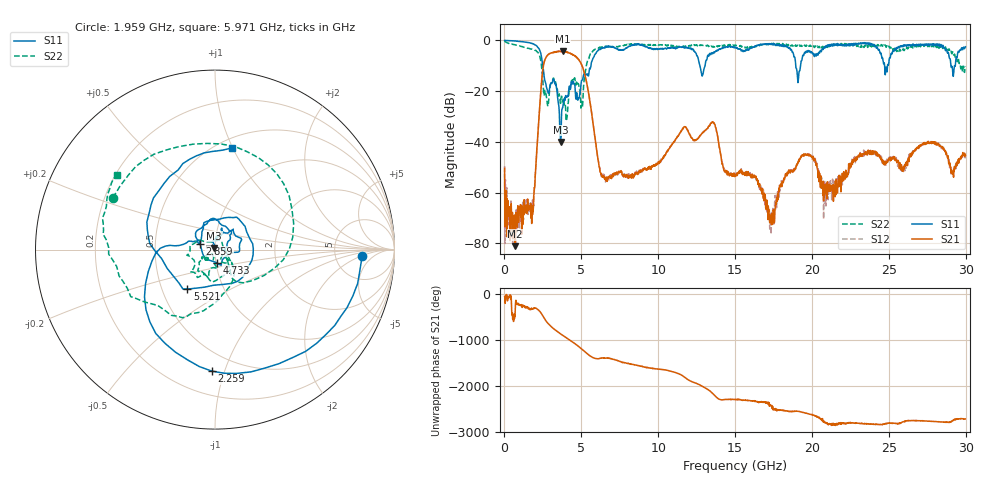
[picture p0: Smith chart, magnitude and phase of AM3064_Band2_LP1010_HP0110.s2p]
# Hz S DB R 50.0
!freq dBS11 angS11 dBS21 angS21 dBS12 angS12 dBS22 angS22
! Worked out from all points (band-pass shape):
!   1600 points, 10 MHz to 29.98 GHz, reference 50 ohm
!   highest |S21| = -4.27 dB at 3.777 GHz (marker M1); lowest = -81.1 dB at 703.5 MHz (marker M2)
!   |S21| within 3 dB of the highest: 2.656 GHz to 4.791 GHz (2.135 GHz wide, 57.3 % of centre)
!   lowest |S11| = -40.1 dB at 3.646 GHz (marker M3), VSWR 1.02, Z = 49.5 + j0.88 ohm
!   |S11| at or under -10 dB: 2.494 GHz to 5.622 GHz (3.129 GHz wide, 77.1 % of centre); 12.71 GHz to 13.05 GHz (331.7 MHz wide, 2.58 % of centre); 18.95 GHz to 19.25 GHz (303.6 MHz wide, 1.59 % of centre)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
!   |S22| runs from -31.2 to -0.3 dB; largest |S21 - S12| = 0.017
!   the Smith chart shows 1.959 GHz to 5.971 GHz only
!   S11 on the Smith chart (normalised r, x): 1.959 GHz: 9.63, -2.16; 2.259 GHz: 0.36, -0.91; 2.859 GHz: 0.84, +0.06; 4.733 GHz: 1.01, -0.15; 5.521 GHz: 0.67, -0.32; 5.971 GHz: 0.59, +0.99
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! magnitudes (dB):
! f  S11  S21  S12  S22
! 10 MHz  0.0  -50.4  -49.5  -0.3
! 703.5 MHz  -0.2  -81.1  -74.6  -1.8
! 1.959 GHz  -1.7  -58.2  -57.9  -3.9
! 2.259 GHz  -3.4  -29.2  -29.1  -5.5
! 2.859 GHz  -20.9  -5.5  -5.6  -24.8
! 3.646 GHz  -40.1  -4.3  -4.3  -24.8
! 3.777 GHz  -26.5  -4.3  -4.3  -24.2
! 4.733 GHz  -22.5  -6.8  -6.8  -16.5
! 5.015 GHz  -15.8  -9.5  -9.5  -24.7
! 5.521 GHz  -11.4  -22.6  -22.6  -6.4
! 5.971 GHz  -4.8  -42.1  -42.1  -3.2
! 6.664 GHz  -2.4  -53.8  -54.5  -2.5
! 10 GHz  -3.4  -48.4  -47.8  -1.8
! 13.54 GHz  -5.3  -32.2  -32.1  -2.6
! 15 GHz  -2.7  -53.6  -53.4  -1.8
! 16.32 GHz  -2.3  -54.1  -53.4  -2.1
! 17.4 GHz  -1.6  -68.2  -68.9  -1.3
! 19.09 GHz  -16.6  -48.0  -47.9  -2.3
! 19.99 GHz  -4.7  -45.8  -46.2  -1.9
! 20.91 GHz  -2.2  -58.0  -65.3  -2.5
! 25 GHz  -9.1  -46.7  -45.9  -2.3
! 29.98 GHz  -2.5  -45.2  -45.9  -10.2
